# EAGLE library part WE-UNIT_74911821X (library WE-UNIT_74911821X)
Off-Line Transformer WE-Unit - Nominal input voltage: 85-265 VAC - Output power 9 W - Operating temperature: -40°C to +125 °C - Clearance and creepage distance 6 mm min. - Isolation voltage 4 kVAC -- Designed for Tiny switch ICs from power integration and NCP101x or 105x of Semiconductor -- Universal input -- Offline-switch mode power supplies
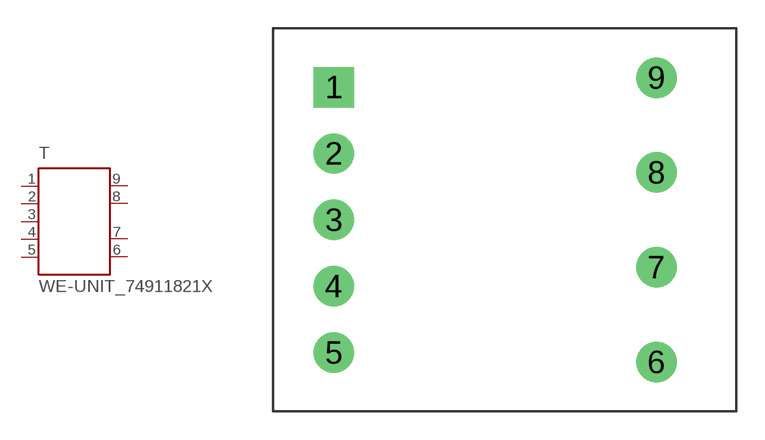
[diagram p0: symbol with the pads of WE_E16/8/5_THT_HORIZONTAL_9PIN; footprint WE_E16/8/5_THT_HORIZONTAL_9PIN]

Designator prefix T

## WE-UNIT_74911821X, WE-UNIT_74911821X-7491182112 (MPN: 7491182112; OC_FARNELL: 1849040; OC_NEWARK: unknown; PACKAGE: E16_8_5; SUPPLIER: Wuerth Elektronik), WE-UNIT_74911821X-7491182124 (MPN: 7491182124; OC_FARNELL: 1849041; OC_NEWARK: 13T9801; PACKAGE: E16_8_5; SUPPLIER: Wuerth Elektronik), WE-UNIT_74911821X-749118215 (MPN: 749118215; OC_FARNELL: 1849039; OC_NEWARK: 13T9802; PACKAGE: E16_8_5; SUPPLIER: Wuerth Elektronik)  [WE_E16/8/5_THT_HORIZONTAL_9PIN]
1  5  pas
2  4  pas
3  3  pas
4  2  pas
5  1  pas
6  9  pas
7  8  pas
8  7  pas
9  6  pas

## Footprint WE_E16/8/5_THT_HORIZONTAL_9PIN (pad centres in mm)
Transformer, E16/8/5 THT Horizontal 9 Pin
drill 1.42 square: 1 -8.5,7
drill 1.42: 2 -8.5,3.5; 3 -8.5,0; 4 -8.5,-3.5; 5 -8.5,-7; 6 8.5,-7.5; 7 8.5,-2.5; 8 8.5,2.5; 9 8.5,7.5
